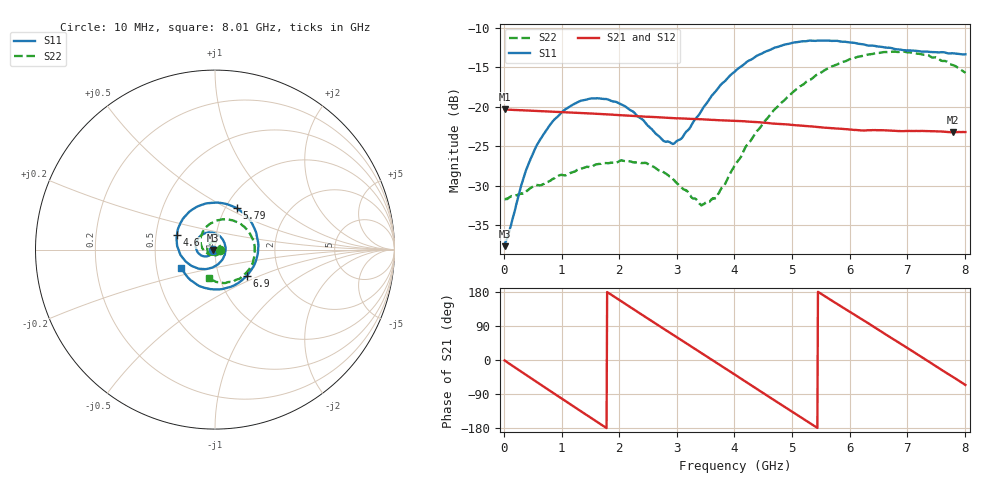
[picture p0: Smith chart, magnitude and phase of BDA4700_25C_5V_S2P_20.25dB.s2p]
!Agilent Technologies,E5071B,MY42404982,A.09.10
!Date: Mon Oct 20 13:36:31 2025
!Data & Calibration Information:
!Freq	S11:SOLT2(ON)	S21:SOLT2(ON)	S12:SOLT2(ON)	S22:SOLT2(ON)
# Hz S RI R 50
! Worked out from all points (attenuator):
!   801 points, 10 MHz to 8.01 GHz, reference 50 ohm
!   highest |S21| = -20.34 dB at 10 MHz (marker M1); lowest = -23.2 dB at 7.8 GHz (marker M2)
!   lowest |S11| = -37.7 dB at 10 MHz (marker M3), VSWR 1.03, Z = 48.7 - j0.151 ohm
!   |S11| at or under -10 dB: start of sweep to end of sweep
!   |S22| runs from -32.5 to -13.0 dB; largest |S21 - S12| = 0.0007
!   S11 on the Smith chart (normalised r, x): 10 MHz: 0.97, -0.00; 4.6 GHz: 0.64, +0.11; 5.79 GHz: 1.13, +0.56; 6.9 GHz: 1.35, -0.42; 8.01 GHz: 0.67, -0.15
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1e7  -0.013 -0.00155  0.0962 -0.00204  0.0962 -0.0022  0.026 -0.000876
3.5e8  -0.0246 -0.027  0.0766 -0.0557  0.0766 -0.0558  0.0222 -0.0177
5.7e8  -0.0429 -0.0377  0.0495 -0.08  0.0494 -0.0801  0.0143 -0.0286
8.8e8  -0.0766 -0.0328  0.000744 -0.0929  0.000703 -0.093  -0.007 -0.0346
1.35e9  -0.1079 0.0189  -0.0664 -0.0625  -0.0665 -0.0625  -0.0366 -0.0176
1.97e9  -0.0527 0.0922  -0.084 0.0283  -0.0841 0.0283  -0.0339 0.0288
2.45e9  0.0262 0.075  -0.0352 0.079  -0.0352 0.0791  -0.00185 0.0441
2.68e9  0.0518 0.0398  -0.00223 0.0857  -0.00217 0.0856  0.0142 0.037
2.96e9  0.0566 -0.0157  0.0369 0.076  0.037 0.0759  0.0265 0.0215
3.44e9  -0.00697 -0.0961  0.0795 0.0244  0.0796 0.0244  0.0182 -0.0154
3.69e9  -0.0669 -0.1081  0.0816 -0.0105  0.0817 -0.0108  -0.000469 -0.0267
4.01e9  -0.1475 -0.079  0.0634 -0.0511  0.0635 -0.0511  -0.0336 -0.0263
4.6e9  -0.2118 0.0823  -0.00976 -0.0781  -0.00971 -0.0782  -0.0791 0.0359
4.92e9  -0.1702 0.1819  -0.048 -0.0605  -0.0479 -0.0607  -0.0725 0.0892
5.35e9  -0.0389 0.2586  -0.0739 -0.0125  -0.0739 -0.0127  -0.015 0.15
5.79e9  0.1226 0.2301  -0.0611 0.0393  -0.0611 0.0394  0.0831 0.1659
6.23e9  0.2275 0.0991  -0.0191 0.068  -0.0185 0.0682  0.1787 0.1097
6.68e9  0.224 -0.0742  0.0328 0.0626  0.0329 0.0627  0.221 -0.00293
6.9e9  0.1765 -0.1461  0.0525 0.0464  0.0526 0.0462  0.2136 -0.0645
7.35e9  0.0208 -0.2223  0.07 -0.00227  0.0701 -0.00245  0.1381 -0.1617
7.8e9  -0.1404 -0.1663  0.0484 -0.049  0.0483 -0.049  0.0169 -0.182
8.01e9  -0.1871 -0.105  0.0283 -0.063  0.0285 -0.0631  -0.0331 -0.1603
